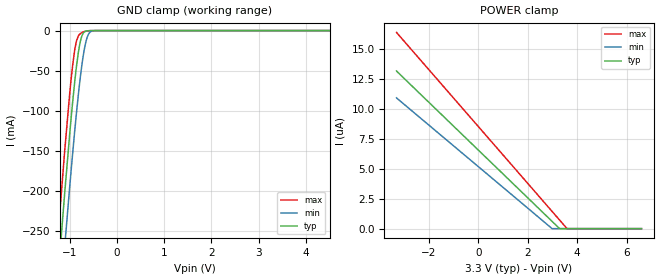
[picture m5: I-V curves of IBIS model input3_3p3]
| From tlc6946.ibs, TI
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|   input3_3p3 Model
[Model]   input3_3p3
Model_type   Input
Vinl = 0.99
Vinh = 2.31
|   typ   min   max
C_comp   1.4847pF   1.4576pF   1.5054pF
|  Where Nom  PVT is Nominal Process, 3.3V,   27C
|   Fast PVT is Strong Process,  3.6V,   -40C
|   Slow PVT is Weak Process,   3.0V,   105C
[Model spec]
|subparameter
Vinl   0.99   0.9   1.08
Vinh   2.31   2.1   2.52
[Voltage Range]   3.3   3   3.6
|Junction Temperature
[Temperature Range]   27   105   -40
[Power Clamp Reference]   3.3   3   3.6
[GND Clamp Reference]   0   0   0
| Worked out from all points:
|   GND clamp passes 1 mA (typ) near -0.67 V on its own axis
[GND Clamp]
|   Voltage   I(typ)   I(min)   I(max)
-3.3V     -1.941A    -1.934A    -1.954A
-1.251V   -312.3mA   -378mA     -260.7mA
-1.211V   -282.2mA   -348.4mA   -230mA
-1.102V   -201.6mA   -268.5mA   -148.8mA
-993.3mV  -125.9mA   -191.8mA   -75.65mA
-933.9mV  -88.15mA   -152.1mA   -42.62mA
-854.7mV  -44.72mA   -102.7mA   -12.96mA
-775.5mV  -14.38mA   -59.36mA   -3.953mA
-716.1mV  -3.663mA   -33.2mA    -1.899mA
-607.2mV  -222.1uA   -5.4mA     -257.2uA
-458.7mV  -5.417uA   -90.58uA   -4.959uA
6.6V      0A         0A         0A
[POWER Clamp]
|   Voltage   I(typ)   I(min)   I(max)
-3.3V     13.19uA    10.94uA    16.42uA
2.977V    625.8nA    16.89nA    1.464uA
3.284V    10.39nA    0A         733nA
3.59V     0A         0A         1.168nA
6.6V      0A         0A         0A
